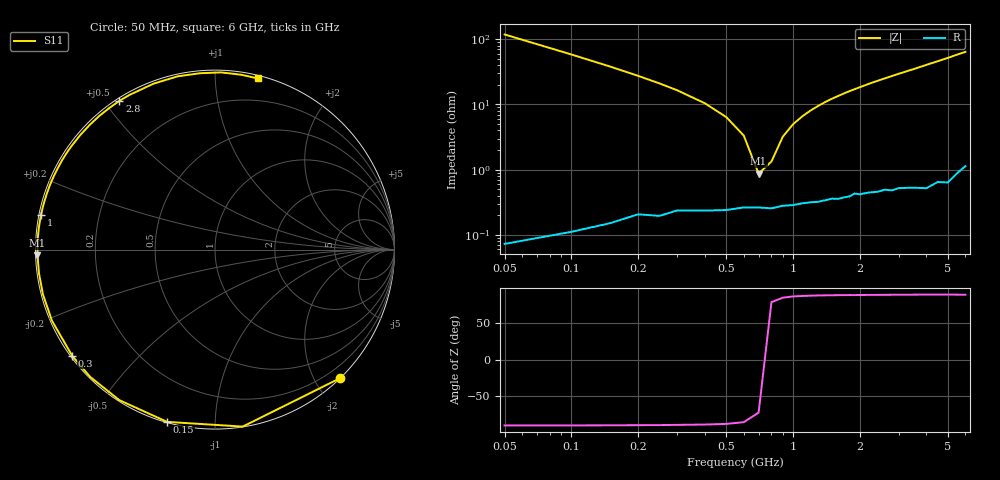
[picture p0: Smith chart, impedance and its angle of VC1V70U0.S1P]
! Infineon Technologies  Discrete & RF Semiconductors
! BBY 56-03
! Si Tuning Diode in SOD323
! VR = 1.75 V
! S-Parameters:  June  1999
# GHz  S  MA  R  50
!  f  S11
! GHz  MAG  ANG
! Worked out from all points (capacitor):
!   34 points, 50 MHz to 6 GHz, reference 50 ohm
!   read as one part to ground: C = 26.8 pF near 50 MHz
!   lowest |Z| = 870 mohm at 700 MHz (marker M1)
!   series resonance near 738.8 MHz, so ESL is about 1.7 nH
!   S11 on the Smith chart (normalised r, x): 50 MHz: 0.00, -2.37; 150 MHz: 0.00, -0.76; 300 MHz: 0.00, -0.33; 1 GHz: 0.01, +0.10; 2.8 GHz: 0.01, +0.55; 6 GHz: 0.02, +1.28
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0.05  0.9996 -45.8
0.1  0.9981 -81.1
0.15  0.9962 -105.5
0.2  0.9937 -122.4
0.25  0.9934 -134.4
0.3  0.9915 -143.4
0.4  0.991 -156.4
0.5  0.9906 -165.4
0.6  0.9896 -172.4
0.7  0.9895 -178.1
0.8  0.9899 177.0
1  0.9887 168.7
1.2  0.9878 161.7
1.3  0.9877 158.5
1.4  0.9871 155.4
1.6  0.9868 149.8
1.8  0.986 144.5
2  0.9853 139.7
2.2  0.9849 135.0
2.4  0.985 130.7
2.8  0.9853 122.7
3  0.9847 118.9
3.5  0.9858 110.3
4  0.9875 102.1
4.5  0.9861 94.7
5  0.9878 88.0
5.5  0.9851 81.5
6  0.983 75.9
